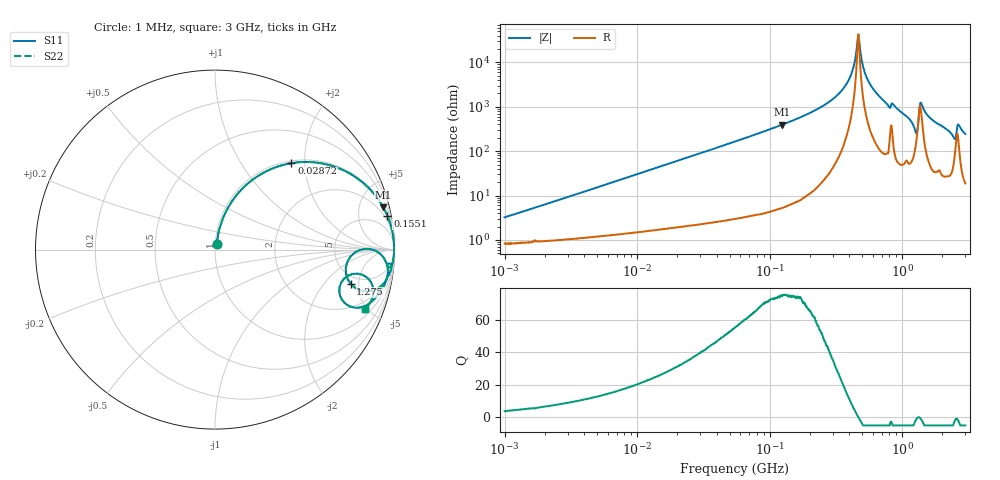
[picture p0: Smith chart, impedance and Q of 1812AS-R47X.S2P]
!s-Parameter Generated by FASTRON Sdn. Bhd.
!FASTRON P/N : 1812AS-R47X
!Keysight Technologies,E4991B,MY54100416,A.01.15
!Date created: Fri Oct 13 15:17:48 2023
!Version  : Rev00 Fri Oct 13 15:17:48 2023
!Data & Calibration Information:
!Freq	S11	S21	S12	S22
!PortZ  Port1:50+j0  Port2:50+j0
!When reading, reference impedance value at option line is always used.
! Remarks : This data is being provided solely for informational purposes.
# Hz S dB R 50
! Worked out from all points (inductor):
!   1601 points, 1 MHz to 3 GHz, reference 50 ohm
!   read as one part in series: L = 497 nH near 1.041 MHz
!   highest Q = 75 at 124.4 MHz (marker M1), where L = 504 nH
!   self-resonance near 466.3 MHz
!   S11 on the Smith chart (normalised r, x): 1 MHz: 1.02, +0.06; 28.72 MHz: 1.04, +1.72; 155.1 MHz: 1, +10; 1.275 GHz: 4.10, -3.97; 3 GHz: 1.37, -4.86
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1000000  -29.87 73.3  -0.08 -1.8  -0.08 -1.8  -29.87 73.3
3804036  -18.78 78.0  -0.15 -6.6  -0.15 -6.6  -18.78 78.0
1.447069e7  -8.11 64.6  -0.87 -23.1  -0.87 -23.1  -8.11 64.6
2.87222e7  -3.84 48.5  -2.51 -40.0  -2.51 -40.0  -3.84 48.5
5.477226e7  -1.44 31.0  -5.76 -57.9  -5.76 -57.9  -1.44 31.0
1.244416e8  -0.30 14.2  -12.22 -75.1  -12.22 -75.1  -0.30 14.2
1.550909e8  -0.18 11.0  -14.38 -78.2  -14.38 -78.2  -0.18 11.0
2.083556e8  -0.09 7.5  -17.74 -81.6  -17.74 -81.6  -0.09 7.5
3.704446e8  -0.02 2.0  -29.23 -84.7  -29.23 -84.7  -0.02 2.0
4.198105e8  -0.02 0.9  -35.91 -81.3  -35.91 -81.3  -0.02 0.9
4.66327e8  -0.02 0.0  -52.55 -7.2  -52.55 -7.2  -0.02 0.0
4.805402e8  -0.02 -0.2  -46.38 60.1  -46.38 60.1  -0.02 -0.2
5.154121e8  -0.02 -0.8  -36.53 79.3  -36.53 79.3  -0.02 -0.8
5.555877e8  -0.03 -1.5  -31.58 82.5  -31.58 82.5  -0.03 -1.5
7.925923e8  -0.14 -5.6  -20.22 78.0  -20.22 78.0  -0.14 -5.6
1.136371e9  -0.31 -10.6  -14.70 73.8  -14.70 73.8  -0.31 -10.6
1.274982e9  -2.16 -14.1  -10.19 37.9  -10.19 37.9  -2.16 -14.1
1.402151e9  -0.41 -4.1  -21.57 54.8  -21.57 54.8  -0.41 -4.1
1.637435e9  -0.27 -10.2  -15.02 75.2  -15.02 75.2  -0.27 -10.2
2.407135e9  -1.34 -22.2  -8.31 57.5  -8.31 57.5  -1.34 -22.2
2.673854e9  -0.96 -12.4  -12.75 56.9  -12.75 56.9  -0.96 -12.4
3e9  -0.90 -21.6  -8.65 64.0  -8.65 64.0  -0.90 -21.6
